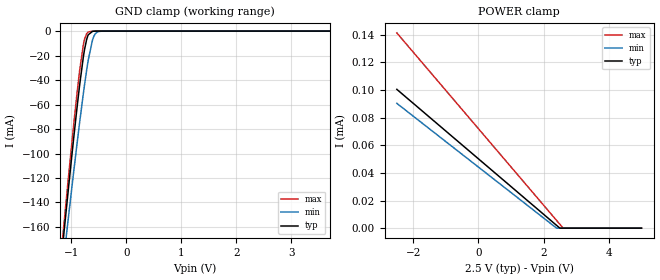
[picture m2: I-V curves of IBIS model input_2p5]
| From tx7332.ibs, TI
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|   input_2p5 Model
[Model]   input_2p5
Model_type   Input
Vinl = 0.625
Vinh = 1.875
|   typ   min   max
C_comp   6.105pF   6.049pF   6.247pF
[Model spec]
|subparameter
Vinl   0.625   0.6   0.65
Vinh   1.875   1.8   1.95
| Where Nom  PVT is Nominal Process, 2.5V, 27C
|   Fast PVT is Strong Process,  2.6V, 0C
|   Slow PVT is Weak Process,   2.4V, 100C
[Voltage Range]   2.5   2.4   2.6
|Junction Temperature
[Temperature Range]   27   100   0
[Power Clamp Reference]   2.5   2.4   2.6
[GND Clamp Reference]   0   0   0
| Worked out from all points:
|   GND clamp passes 1 mA (typ) near -0.64 V on its own axis
[GND Clamp]
|   Voltage   I(typ)   I(min)   I(max)
-2.5V     -801mA     -750.2mA   -829.3mA
-1.173V   -180.9mA   -198.9mA   -174.7mA
-1.075V   -137.5mA   -160.1mA   -129mA
-955mV    -85.82mA   -113.5mA   -74.84mA
-850mV    -43.91mA   -74.4mA    -32.08mA
-767.5mV  -16.7mA    -45.88mA   -7.844mA
-722.5mV  -6.755mA   -31.81mA   -2.055mA
-692.5mV  -2.973mA   -23.36mA   -715.8uA
-595mV    -110.9uA   -4.677mA   -39.67uA
-542.5mV  -25.11uA   -1.251mA   -19.32uA
-467.5mV  -10.2uA    -151.4uA   -13.27uA
5V        0A         0A         0A
[POWER Clamp]
|   Voltage   I(typ)   I(min)   I(max)
-2.5V     100.4uA    90.27uA    141.2uA
2.39V     2.145uA    115.7nA    5.753uA
2.495V    34.73nA    0A         2.844uA
2.592V    0A         0A         143.1nA
5V        0A         0A         0A
